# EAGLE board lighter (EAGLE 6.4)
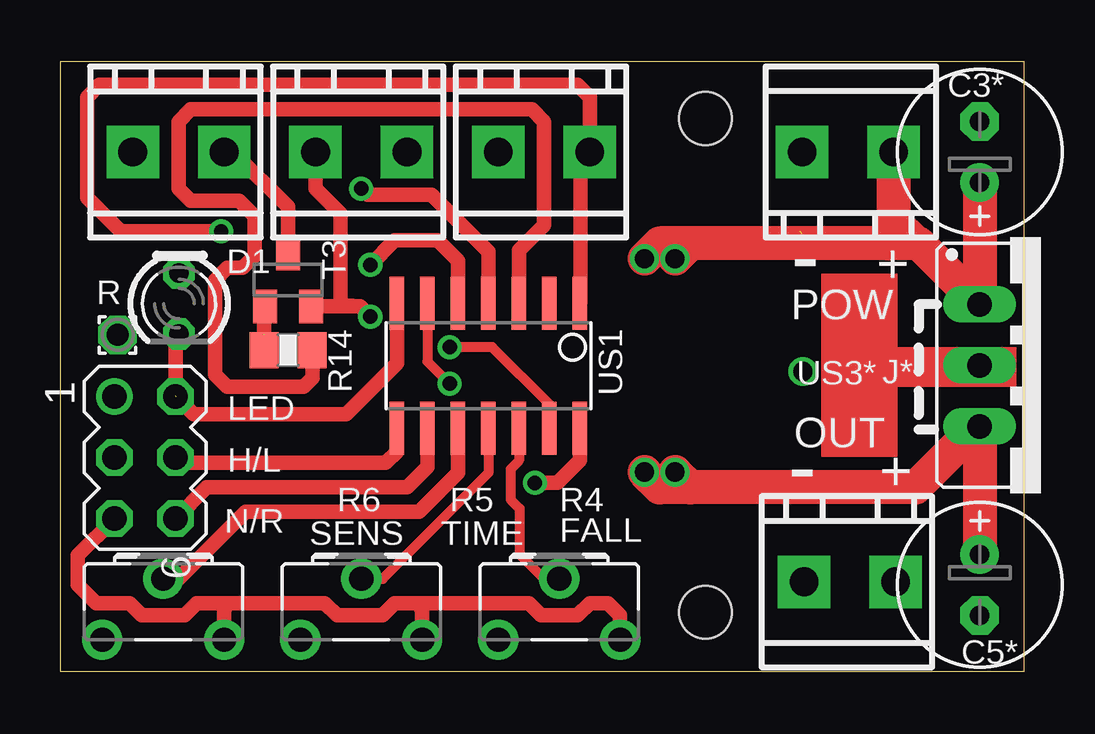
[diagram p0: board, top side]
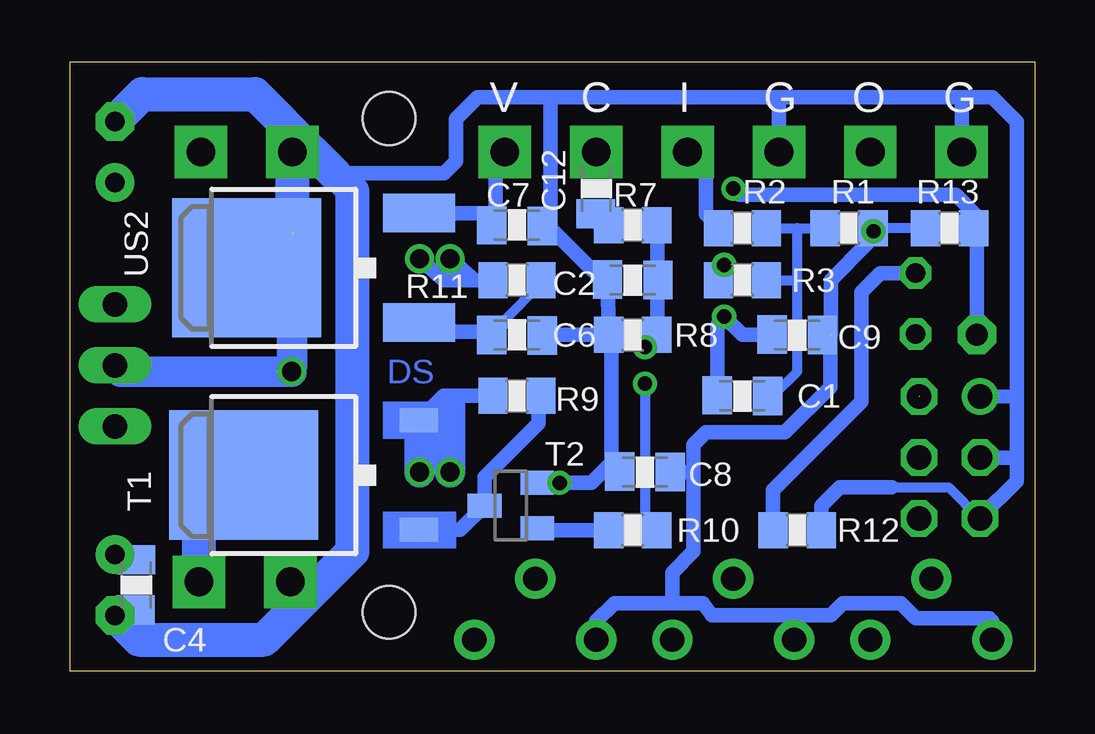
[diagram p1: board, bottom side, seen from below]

Size 40.19 x 25.38 mm. Coordinates in mm from the lower left corner, seen from the top.
Outline: 0,0 40.19,0 40.19,25.38 0,25.38 0,0
Copper layers (1*16): Top 0.035mm / dielectric 1.5mm / Bottom 0.035mm
Design rules "default": minimum track width 10mil, minimum drill 24mil, track to track 8mil, track to pad 8mil, pad to pad 8mil, via to via 8mil, smd to smd 8mil, copper to edge 40mil, drill to drill 8mil, minimum pad ring 10mil, minimum via ring 8mil, stop-mask expansion 4mil, vias tented up to drill 0mil, thermal gap 10mil
Holes 2.2 mm at 26.91,2.45 26.91,23.02

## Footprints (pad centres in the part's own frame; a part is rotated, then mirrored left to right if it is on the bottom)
C0805K = smd 1.219 x 1.6: 1 -1.051,0; 2 1.051,-0.025
E2,5-7 = drill 0.813 pad 1.6: + -1.27,0 | drill 0.813 pad 1.6 octagon: - 1.27,0
ARK2/300 = drill 1.2 pad 2.184 square: 1 -2.54,0; 2 1.27,0
LED3MM = drill 0.813 octagon: A -1.27,0; K 1.27,0
MA03-2 = drill 1.016: 1 -2.54,-1.27 | drill 1.016 octagon: 2 -2.54,1.27; 3 0,-1.27; 4 0,1.27; 5 2.54,-1.27; 6 2.54,1.27
R0805 = smd 1.219 x 1.5: 1 -1.001,0; 2 1.001,0
CA6H = drill 1.016 pad 1.676: A -2.54,0; E 2.54,0; S 0,2.54
1,6/0,9 = drill 0.914 pad 1.6 octagon: 1 0,0
TO252 = smd 1 x 1.6: 1 -2.28,-4.8; 2 2.28,-4.8 | smd 5.4 x 6.2: 3 0,2.5
SOT23 = smd 1 x 1.4: 1 -0.95,-1.1; 2 0.95,-1.1; 3 0,1.1
SOIC14 = smd 0.61 x 2.21: 1 -3.81,-2.603; 2 -2.54,-2.603; 3 -1.27,-2.603; 4 0,-2.603; 5 1.27,-2.603; 6 2.54,-2.603; 7 3.81,-2.603; 8 3.81,2.603; 9 2.54,2.603; 10 1.27,2.603; 11 0,2.603; 12 -1.27,2.603; 13 -2.54,2.603; 14 -3.81,2.603
DPACK = smd 1.6 x 3: 1 -2.28,-4.8; 3 2.28,-4.8 | smd 5.8 x 6.2: 4 0,2.38
78XXS = drill 1.016 long: GND 0,-2.54; IN -2.54,-2.54; OUT 2.54,-2.54

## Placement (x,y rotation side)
C1  100nF  [C0805K]  12.18,11.46 180 bottom
C2  18pF  [C0805K]  16.75,16.29 180 bottom
C3*  220uF  [E2,5-7]  38.34,21.62 90 top
C4  100nF  [C0805K]  37.45,3.59 270 bottom
C5*  220uF  [E2,5-7]  38.34,3.59 270 top
C6  100nF  [C0805K]  21.58,14 0 bottom
C7  100nF  [C0805K]  21.58,18.58 0 bottom
C8  10uF  [C0805K]  16.24,8.29 180 bottom
C9  10uF  [C0805K]  9.89,14 180 bottom
C12  100pF  [C0805K]  18.27,20.1 270 bottom
CON1  [ARK2/300]  13.19,21.62 0 top
CON2  [ARK2/300]  20.81,21.62 0 top
CON3  [ARK2/300]  33.56,3.72 0 top
CON4  [ARK2/300]  32.21,21.62 180 top
CON5  [ARK2/300]  5.57,21.62 0 top
D1  LED  [LED3MM]  4.96,15.31 270 top
PROG  [MA03-2]  3.55,8.89 270 top
R1  15k  [R0805]  7.73,18.45 0 bottom
R2  2.2k  [R0805]  12.18,18.45 0 bottom
R3  15k  [R0805]  12.18,16.29 180 bottom
R4  20k  [CA6H]  20.81,1.3 0 top
R5  20k  [CA6H]  12.56,1.3 0 top
R6  20k  [CA6H]  4.3,1.3 0 top
R7  2.2k  [R0805]  16.75,18.58 180 bottom
R8  470k  [R0805]  16.75,14 180 bottom
R9  2.2k  [R0805]  21.58,11.46 180 bottom
R10  2.2k  [R0805]  16.75,5.87 180 bottom
R11  20R  [R0805]  21.58,16.29 0 bottom
R12  2.2k  [R0805]  9.89,5.87 180 bottom
R13  2.2k  [R0805]  3.54,18.45 0 bottom
R14  15k  [R0805]  9.51,13.37 180 top
RST  [1,6/0,9]  2.4,14 0 top
T1  IRLR9343  [TO252]  30.47,8.16 90 bottom
T2  PMBT2222  [SOT23]  21.83,6.89 90 bottom
T3  2N2222  [SOT23]  9.51,16.29 0 top
US1  TINY24/44  [SOIC14]  17.86,12.71 180 top
US2  78M05  [DPACK]  30.47,16.8 90 bottom
US3*  7812  [78XXS]  40.88,12.73 270 top

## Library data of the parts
C1 C2 C3* C4 C5* C6-C9 C12 R1-R3 R7-R14 = rcl
CON1-CON5 = ds_lib_eagle
D1 = led
PROG = con-lstb; OC_FARNELL: unknown; OC_NEWARK: unknown
R4-R6 = pot
RST = wirepad
T1 = transistor-fet
T2 T3 = transistor-npn
US1 = avr-4
US2 US3* = v-reg

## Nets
C: C12.1 CON2.1
CAP: C2.1 R7.1 R8.1 US1.13
CF1: PROG.4 US1.8
CF2: PROG.6 US1.9
DRV: R10.1 US1.6
EXT: R14.1 US1.3
GND: C1.2 C2.2 C3*.- C4.2 C5*.- C6.2 C7.2 C8.2 C9.2 CON1.1 CON3.1 CON4.2 CON5.1 PROG.1 PROG.3 PROG.5 R4.E R5.E R6.E R8.2 R12.1 T2.2 T3.2 US1.14 US2.4 US3*.GND
I: CON1.2 R2.1
IN: R3.2 US1.5
LED: D1.K PROG.2 US1.7
N$1: D1.A R12.2
N$2: R9.1 T1.1 T2.3
N$3: R10.2 T2.1
N$4: C1.1 R1.1 R2.2 R3.1
N$5: C12.2 R7.2
N$6: R14.2 T3.1
N$7: CON5.2 T3.3
N$9: C6.1 R11.2 US2.1
OUT: CON3.2 T1.3
RST: R13.2 RST.1 US1.4
V1: R4.S US1.12
V2: R5.S US1.11
V3: R6.S US1.10
V+: C3*.+ CON4.1 R11.1 US3*.IN
VCC: C4.1 C5*.+ R9.2 T1.2 US3*.OUT
VDD: C7.1 C8.1 C9.1 CON2.2 R1.2 R4.A R5.A R6.A R13.1 US1.1 US2.3

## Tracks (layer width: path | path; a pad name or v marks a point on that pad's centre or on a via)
C
  Bottom 0.406: CON2.1 C12.1
CAP  (via drill 0.6)
  Top 0.406: US1.13 20.4,11.12 18.02,13.49 v16.24,13.49
  Bottom 0.406: v16.24,13.49 15.86,13.94 R8.1
  Bottom 0.61: R7.1 C2.1 R8.1
CF1
  Top 0.61: PROG.4 5.1,8.67 13.57,8.67 14.05,9.14 US1.8
CF2
  Top 0.61: US1.9 15.32,8.51 14.46,7.65 6.12,7.65 PROG.6
DRV  (via drill 0.6)
  Top 0.406: US1.6 15.32,12.89 v16.24,11.97
  Bottom 0.406: v16.24,11.97 16.24,6.32 R10.1
EXT
  Top 0.61: US1.3 19.13,17.52 20.18,18.58 20.18,22.89 19.67,23.4 5.45,23.4 4.94,22.89 4.94,20.1 5.45,19.59 7.48,19.59 8.11,18.96 8.11,17.3 7.61,16.8 6.97,16.8 6.46,16.29 6.46,12.35 6.97,11.84 10.15,11.84 10.53,12.22 10.53,13.49 R14.1
GND  (via drill 0.6, 0.8)  (1 unrouted)
  Top 0.61: R4.E 23.35,2.32 22.85,2.83 22.08,2.83 21.58,2.32 20.05,2.32 19.54,2.83 14.97,2.83 | 14.97,2.83 13.96,2.83 13.45,2.32 11.54,2.32 11.04,2.83 6.97,2.83 | 6.97,2.83 5.7,2.83 5.19,2.32 3.41,2.32 2.91,2.83 1.51,2.83 0.75,3.59 0.75,4.82 PROG.5 | R6.E 6.84,2.45 6.97,2.83 | R5.E 15.1,2.45 14.97,2.83 | CON1.1 10.65,20.1 11.69,19.06 11.69,15.25 12.52,15.19 | US1.14 21.67,8.78 T2.2 v19.8,7.84 | T3.2 12.52,15.19 | 12.52,15.19 v12.94,14.76
  Bottom 0.406: 5.96,7.65 3.58,7.65 PROG.5 | US2.4 30.85,16.8 30.85,18.32 | C8.2 17.64,8.31 17.64,8.67 | C7.2 20.31,18.55 20.31,18.58 20.18,18.58 20.18,18.7
  Bottom 0.61: R8.2 C2.2 18.08,16.67 18.4,16.67 20.31,18.58 | 3.03,23.91 1.76,23.91 0.75,22.89 0.75,11.44 | 3.03,23.91 10.65,23.91 | 10.65,23.91 20.18,23.91 | 20.18,23.91 23.23,23.91 24.12,23.02 24.12,21.24 24.62,20.73 29.2,20.73 | T2.2 v19.8,7.84 18.47,7.84 17.64,8.67 17.64,13.94 R8.2 | C5*.- 37.39,2.32 C4.2 | CON1.1 10.65,23.91 | 0.75,11.44 PROG.1 | PROG.5 2.28,6.38 0.75,7.91 0.75,8.8 | 0.75,8.8 0.75,11.44 | PROG.3 0.84,8.89 0.75,8.8 | C1.2 13.23,14.42 v12.94,14.76 12.18,14 10.94,14 C9.2 | 20.18,18.51 20.18,18.7 20.18,23.91 | CON5.1 3.03,23.91 | R12.1 8.89,6.88 8.11,7.65 5.96,7.65 | R8.2 20.52,14 C6.2
  Bottom 1.27: CON3.1 29.7,3.72 | 28.43,19.97 30.02,21.56 30.08,21.62 CON4.2 | 30.94,18.2 30.94,12.77 v30.97,12.48 38.09,12.48 US3*.GND
  Bottom 1.422: 28.43,19.97 28.43,4.99 29.7,3.72 32.12,1.3 37.32,1.3 C5*.- | CON4.2 30.94,18.2 | C3*.- 37.2,24.04 32.5,24.04 30.08,21.62 | 29.2,20.73 30.02,21.56
I
  Bottom 0.61: CON1.2 14.34,21.62 13.7,20.99 13.7,19.02 R2.1
IN  (via drill 0.6)
  Top 0.61: US1.5 16.59,17.09 15.73,17.94 13.96,17.94 v12.94,16.92
  Bottom 0.61: v12.94,16.92 12.94,16.48 R3.2
LED  (1 unrouted)
  Top 0.61: 4.96,13.98 D1.K 4.82,13.89 PROG.2 | 4.81,11.46 5.57,10.7 11.92,10.7 14.05,12.83 US1.7
N$1
  Bottom 0.61: D1.A 6.43,16.58 7.22,15.78 7.22,11.21 10.91,7.53 10.91,5.89 R12.2
N$2
  Bottom 0.61: T1.1 23.94,5.88 T2.3 22.93,8.08 20.69,10.32 20.69,11.4 R9.1
N$3
  Bottom 0.61: R10.2 20.66,5.87 T2.1
N$4
  Bottom 0.406: 10.91,11.46 9.89,12.48 9.89,16.29 | 9.89,16.29 9.89,18.45 | 9.89,18.45 R1.1 | R2.2 9.89,18.45 | R3.1 9.89,16.29
  Bottom 0.61: C1.1 10.91,11.46
N$5
  Bottom 0.406: C12.2 R7.2
N$6
  Top 0.61: R14.2 8.51,15.52 T3.1
N$7
  Top 0.61: CON5.2 7.22,21.62 9.51,19.34 T3.3
N$9
  Bottom 0.406: R11.2 20.63,16.1 22.08,14.64 22.08,14.44 C6.1
  Bottom 0.61: C6.1 22.53,14.06 22.59,14.13 25.28,14.13 US2.1
OUT
  Bottom 1.27: 34.83,6.29 T1.3
  Bottom 1.422: CON3.2 34.83,6.29
RST  (via drill 0.6)
  Top 0.61: US1.4 17.86,17.47 15.48,19.84 12.81,19.84 v12.56,20.1
  Bottom 0.406: 2.4,18.96 R13.2
  Bottom 0.61: v12.56,20.1 12.3,19.84 3.29,19.84 2.4,18.96 RST.1
V1
  Top 0.406: US1.12 19.13,8.76 18.78,8.42 18.78,7.14 19.16,6.76 19.16,4.86 20.18,3.84 R4.S
V2
  Top 0.406: US1.11 17.86,8.25 13.45,3.84 R5.S
V3
  Top 0.61: US1.10 16.59,8.25 14.97,6.64 7.73,6.64 4.94,3.84 R6.S
V+  (via drill 0.8)
  Top 1.27: 34.75,18.86 35.8,17.81
  Top 1.422: CON4.1 34.75,18.86 | C3*.+ US3*.IN 35.8,17.81 34.53,17.81 | 34.53,17.81 26.27,17.81 v25.64,17.18 | v24.37,17.18 25,17.81 34.53,17.81
  Bottom 0.61: v25.64,17.18 24.62,16.29 23.35,16.29 | 22.46,16.29 R11.1 23.35,16.29 | v24.37,17.18 23.35,16.29
VCC  (via drill 0.8)
  Top 1.27: US3*.OUT 37.96,9.94
  Top 1.422: US3*.OUT C5*.+ | 37.96,9.94 35.67,7.65 26.27,7.65 | 26.27,7.65 v25.64,8.29 | v24.37,8.29 25,7.65 26.27,7.65
  Bottom 0.61: R9.2 24.64,11.46 T1.2 25.67,10.35 25.64,10.32 | C5*.+ 37.39,4.86 C4.1
  Bottom 1.27: v25.64,8.29 25.64,10.32 | v24.37,8.29 24.37,11.08
VDD  (via drill 0.6)  (1 unrouted)
  Top 0.61: US1.1 21.7,15.35 21.7,21.24 CON2.2 22.08,23.91 21.58,24.42 1.64,24.42 1.13,23.91 1.13,19.72 2.53,18.32 v6.72,18.32
  Bottom 0.406: 10.02,2.32 10.02,2.19 10.15,2.32 | 1.76,2.06 1.89,2.19 | R13.1 R1.2 6.97,18.19 6.91,18.13 v6.72,18.32 | 8.52,14 8.52,14.64
  Bottom 0.61: US2.3 23.03,19.08 C7.1 22.46,18.64 22.46,21.24 CON2.2 | R5.A 10.02,2.19 | R6.A 1.76,2.06 | 1.89,2.19 4.94,2.19 5.57,2.83 7.99,2.83 8.5,2.32 10.02,2.32 | R4.A 18.27,2.06 17.51,2.83 15.1,2.83 | 15.1,2.83 13.83,2.83 13.45,2.32 10.15,2.32 | 14.21,8.29 14.74,8.31 C8.1 14.21,8.29 | 14.21,8.29 14.21,4.99 15.1,4.1 15.1,2.83 | C9.1 8.52,14 8.52,13.9 8.52,11.82 10.4,9.94 13.7,9.94 14.21,9.43 14.21,8.29 | 6.97,18.19 6.97,17.81 8.5,16.29 8.5,14
(copper drawn outside any net)
  shapes: Bottom area x2, Top area x2

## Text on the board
Bottom: DS
tPlace: - | + | R | POW | J* | LED | OUT | H/L | + | - | N/R | SENS | TIME | FALL
bPlace: G | O | G | I | C | V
